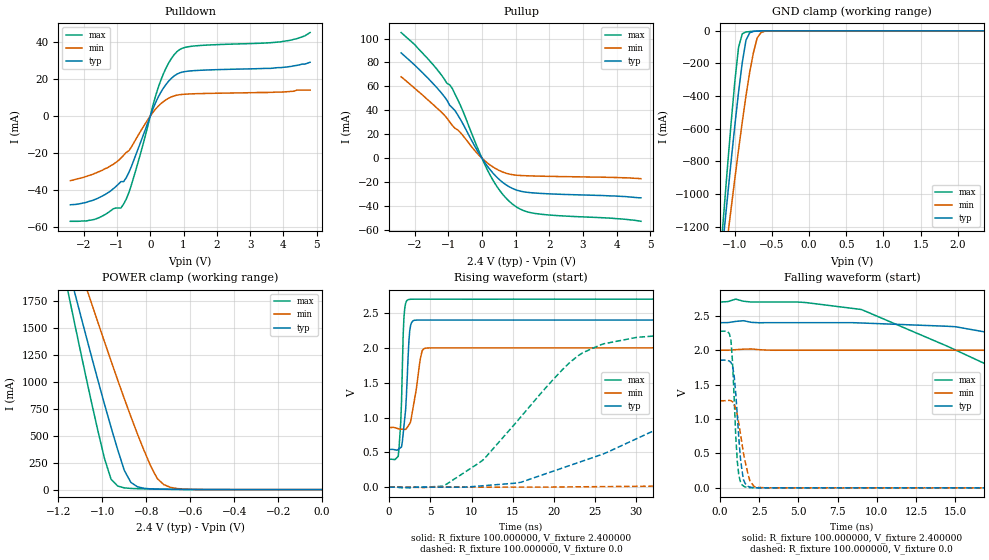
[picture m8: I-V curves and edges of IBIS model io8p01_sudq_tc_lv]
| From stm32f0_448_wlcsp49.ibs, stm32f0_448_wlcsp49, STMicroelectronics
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|   Model io8p01_sudq_tc_lv
[Model]  io8p01_sudq_tc_lv
Model_type I/O
Polarity   Non-Inverting
Enable   Active-Low
Vinl =   0.720000V
Vinh =   1.680000V
Vmeas =  1.200000V
Cref =   50.000000pF
Rref =   100.000000M
Vref =   0.0V
C_comp   1.378000pF   1.292700pF   1.486400pF
[Temperature Range]   25.000000   0.125000k   -40.000000
[Pullup Reference]   2.400000V   2.000000V   2.700000V
[Pulldown Reference]   0.0V   0.0V   0.0V
[POWER Clamp Reference]   2.400000V   2.000000V   2.700000V
[GND Clamp Reference]   0.0V   0.0V   0.0V
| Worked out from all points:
|   slope of the pulldown table from 0 to 0.36 V, typ, clamps not added: 25.7 ohm
|   slope of the pullup table from 0 to 0.36 V, typ, clamps not added: 26.8 ohm
|   GND clamp passes 1 mA (typ) near -0.67 V on its own axis
|   POWER clamp passes 1 mA (typ) near -0.60 V on its own axis
|   rising waveform, R_fixture 100.000000, V_fixture 2.400000: 20-80 % time 540ps typ, 871ps min, 354ps max; typ from 0.542 V to 2.4 V
|   rising waveform, R_fixture 100.000000, V_fixture 0.0: 20-80 % time 22.5ns typ, 61.8ns min, 10.3ns max; typ from 0 V to 1.85 V
|   falling waveform, R_fixture 100.000000, V_fixture 2.400000: 20-80 % time 28.7ns typ, 66.4ns min, 14.7ns max; typ from 2.4 V to 0.542 V
|   falling waveform, R_fixture 100.000000, V_fixture 0.0: 20-80 % time 377ps typ, 594ps min, 284ps max; typ from 1.85 V to 0 V
[Pulldown]
|Voltage   I(typ)   I(min)   I(max)
-2.4V     -47.8mA    -34.8mA    -56.7mA
-1.68V    -45.1mA    -31mA      -55.7mA
-1.12V    -39.3mA    -26.1mA    -50.05mA
-800mV    -35.33mA   -21.13mA   -47.42mA
-640mV    -30.33mA   -18.65mA   -41.16mA
-480mV    -23.12mA   -14mA      -31.94mA
240mV     10.22mA    5.339mA    15.38mA
480mV     17.22mA    8.864mA    26.1mA
800mV     22.59mA    11.27mA    34.68mA
1.36V     24.54mA    12.05mA    37.84mA
3.92V     26.1mA     12.9mA     40mA
4.8V      29mA       14mA       45mA
[Pullup]
|Voltage   I(typ)   I(min)   I(max)
-2.4V     88mA       68mA       105mA
-2V       77.9mA     58.5mA     95mA
-1.36V    59.6mA     42.5mA     75.1mA
-880mV    42.12mA    27.44mA    58.22mA
-560mV    28.45mA    18.75mA    39mA
-160mV    7.44mA     4.66mA     10.64mA
160mV     -6.607mA   -3.947mA   -9.704mA
480mV     -16.91mA   -9.806mA   -25.1mA
880mV     -24.9mA    -13.63mA   -37.75mA
1.2V      -27.87mA   -14.5mA    -43.37mA
1.6V      -29.13mA   -14.89mA   -46.24mA
4.72V     -33.1mA    -17.1mA    -52.7mA
[GND_clamp]
|Voltage   I(typ)   I(min)   I(max)
-2.4V     -7.358A    -6.372A    -8.78A
-1.2V     -1.489A    -1.65A     -1.416A
-1.15V    -1.254A    -1.461A    -1.124A
-1.1V     -1.024A    -1.273A    -838.2mA
-1.05V    -797.6mA   -1.088A    -563.1mA
-950mV    -374.6mA   -728.7mA   -100.8mA
-900mV    -194.3mA   -557.9mA   -18.01mA
-850mV    -56.94mA   -397.4mA   -7.08mA
-750mV    -3.582mA   -133.8mA   -2.771mA
-700mV    -1.516mA   -44.7mA    -1.516mA
-600mV    -235.4uA   -2.939mA   -209.5uA
2.35V     0A         0A         0A
[POWER_clamp]
|Voltage   I(typ)   I(min)   I(max)
-2.4V     9.979A     9.967A     9.901A
-1.17V    2.182A     2.481A     1.978A
-1.14V    1.945A     2.294A     1.683A
-1.11V    1.71A      2.108A     1.391A
-1.08V    1.476A     1.923A     1.102A
-1.05V    1.245A     1.739A     819.9mA
-960mV    578.2mA    1.196A     96.06mA
-900mV    179.5mA    846.7mA    16.04mA
-870mV    67.18mA    678.8mA    10.82mA
-780mV    6.749mA    219.9mA    5.853mA
-720mV    3.355mA    46.34mA    3.808mA
0V        0A         0A         0A
[Ramp]
| variable   typ   min   max
dV/dt_r  1.11318/22.44200n   0.75678/61.87164n   1.36560/10.33061n
dV/dt_f  1.11505/28.61514n   0.68783/66.49225n   1.37972/14.71732n
R_load = 100.000000
[Rising Waveform]
R_fixture= 100.000000
V_fixture= 2.400000
V_fixture_min= 2.000000
V_fixture_max= 2.700000
|time   V(typ)   V(min)   V(max)
0s        541.6mV    855mV      400.5mV
1.101ns   541.5mV    839.4mV    442.8mV
1.401ns   568.2mV    832.4mV    919.3mV
1.802ns   882.4mV    829.4mV    2.451V
2.002ns   1.114V     827.9mV    2.638V
2.302ns   1.872V     876.8mV    2.692V
2.703ns   2.357V     1.003V     2.698V
3.804ns   2.4V       1.853V     2.699V
4.404ns   2.4V       1.995V     2.699V
49.85ns   2.4V       2V         2.7V
[Rising Waveform]
R_fixture= 100.000000
V_fixture= 0.0
V_fixture_min= 0.0
V_fixture_max= 0.0
|time   V(typ)   V(min)   V(max)
0s        804.5pV    13.47nV    619.4pV
6.507ns   -400.5uV   -184uV     13.44mV
11.01ns   16.31mV    -168uV     355.3mV
23.52ns   375.5mV    5.097mV    1.931V
38.04ns   1.124V     66.07mV    2.224V
49.55ns   1.596V     164.7mV    2.255V
63.56ns   1.765V     309.1mV    2.272V
111.1ns   1.849V     924.6mV    2.276V
138.6ns   1.855V     1.129V     2.276V
249.2ns   1.855V     1.266V     2.276V
[Falling Waveform]
R_fixture= 100.000000
V_fixture= 2.400000
V_fixture_min= 2.000000
V_fixture_max= 2.700000
|time   V(typ)   V(min)   V(max)
0s        2.4V       2V         2.7V
9.009ns   2.396V     2V         2.592V
15.02ns   2.341V     2V         2.003V
28.03ns   1.808V     1.956V     814.3mV
33.53ns   1.558V     1.925V     580.4mV
40.04ns   1.291V     1.873V     492mV
55.56ns   815mV      1.669V     428.3mV
73.57ns   628.4mV    1.447V     407.7mV
126.1ns   550.2mV    1.016V     400.4mV
249.2ns   541.6mV    855mV      400.5mV
[Falling Waveform]
R_fixture= 100.000000
V_fixture= 0.0
V_fixture_min= 0.0
V_fixture_max= 0.0
|time   V(typ)   V(min)   V(max)
0s        1.855V     1.266V     2.276V
700.7ps   1.823V     1.265V     2.141V
900.9ps   1.63V      1.209V     1.32V
1.101ns   1.06V      1.063V     390.9mV
1.201ns   720.7mV    934.5mV    181.2mV
1.401ns   253.5mV    642.6mV    46.34mV
1.702ns   35.88mV    284.7mV    7.383mV
2.202ns   3.105mV    15.08mV    668uV
2.903ns   237.1uV    2.061mV    333.1uV
49.85ns   804.5pV    13.47nV    619.4pV
